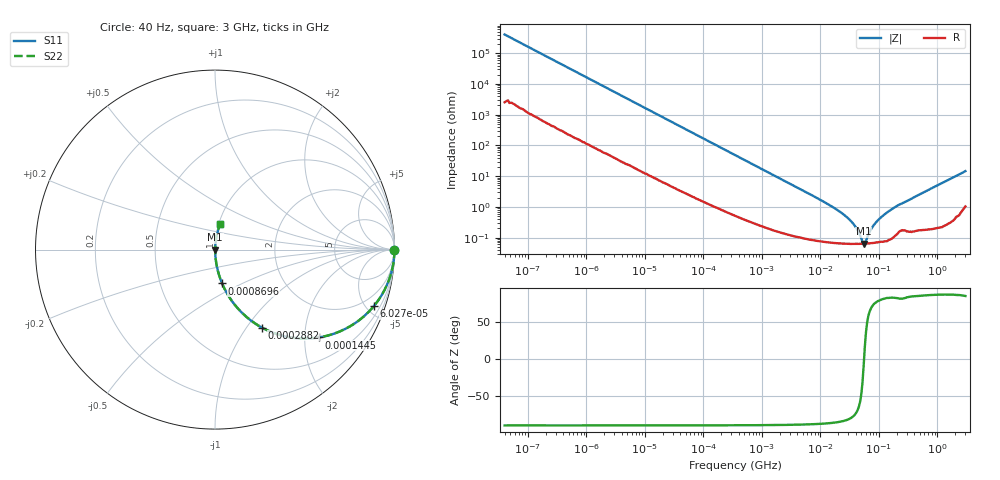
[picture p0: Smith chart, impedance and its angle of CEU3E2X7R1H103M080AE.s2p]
! S-parameter Generated by TDK Corporation
! Copyright(C) 2015 TDK Corporation.
! All Rights Reserved.
! TDK P/N: CEU3E2X7R1H103M080AE (Multilayer Ceramic Chip Capacitors)
! Property: C=10nF
! Size(LxWxT): 1.6x0.8x0.8mm, 0.063x0.031x0.031inches
! Model Type: s2p (Touchstone File Format Version 1.0)
! Frequency: DC=Yes Start=0.00004MHz Stop=3000MHz 396points Log-sweep
! Note: This model was converted from impedance.
! Model Generated on Jun. 23, 2015
! Hash(MD5):
! Port Assignments:
!  1 ---| |--- 2
! Applicable Conditions:
!  Temperature = 25 degC
!  DC Bias Voltage = 0 V
!  Small Signal Operation
! Terms and conditions regarding TDK Simulation Models
! (1)This simulation model is being provided solely for informational purposes. Please refer to the specifications of the products in terms of detailed characteristics of such products.
! (2)In no event shall TDK Corporation of any of its subsidiaries be liable for any loss or damage arising, directly or indirectly,
!  From any information contained in this simulation model, including, but not limited to loss or damages arising from any inaccuracies, omissions or errors in connection with such information.
! (3)Any and all copyrights on this simulation model are owned by TDK Corporation.
!  Duplication or redistribution of this simulation model without prior written permission from TDK Corporation is prohibited.
! (4)This simulation model is subject to any modification or change without any prior notice.
! (5)Neither TDK Corporation nor any of its subsidiaries shall make any warranty, express or implied,
!  Including but not limited to the correctness, implied warranties of merchantability and fitness for a particular purpose with respect to this simulation models.
! (6)The use of this simulation model shall be deemed to have consented to the terms and conditions hereof.
# MHz S MA R 50
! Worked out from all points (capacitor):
!   395 points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, 40 Hz to 3 GHz, reference 50 ohm
!   read as one part in series: C = 9.76 nF near 41.88 Hz
!   lowest |Z| = 64.2 mohm at 54.73 MHz (marker M1)
!   series resonance near 55.61 MHz, so ESL is about 840 pH
!   S11 on the Smith chart (normalised r, x): 40 Hz: open; 60.27 kHz: 1.05, -5.60; 144.5 kHz: 1.02, -2.35; 288.2 kHz: 1.01, -1.18; 869.6 kHz: 1.01, -0.39; 3 GHz: 1.02, +0.29
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4e-05  1 -0.0  0.0002442 89.6  0.0002442 89.6  1 -0.0
0.000834128  1 -0.3  0.005044 89.3  0.005044 89.3  1 -0.3
0.01739424  0.9939 -5.9  0.103 83.7  0.103 83.7  0.9939 -5.9
0.06026525  0.9393 -19.6  0.3353 69.9  0.3353 69.9  0.9393 -19.6
0.09119145  0.8771 -28.2  0.4728 61.3  0.4728 61.3  0.8771 -28.2
0.144487  0.7577 -40.2  0.6458 49.3  0.6458 49.3  0.7577 -40.2
0.2881647  0.5065 -59.0  0.8571 30.4  0.8571 30.4  0.5065 -59.0
0.3464102  0.4397 -63.3  0.8936 26.1  0.8936 26.1  0.4397 -63.3
0.8696408  0.193 -78.1  0.9787 11.1  0.9787 11.1  0.193 -78.1
2.183178  0.07862 -84.5  0.9955 4.5  0.9955 4.5  0.07862 -84.5
7.22376  0.02371 -86.6  0.9989 1.4  0.9989 1.4  0.02371 -86.6
18.13479  0.008661 -85.1  0.9993 0.5  0.9993 0.5  0.008661 -85.1
30.08671  0.004173 -81.1  0.9994 0.2  0.9994 0.2  0.004173 -81.1
41.52283  0.001972 -71.4  0.9994 0.1  0.9994 0.1  0.001972 -71.4
54.72828  0.0006419 -8.8  0.9994 0.0  0.9994 0.0  0.0006419 -8.8
57.30589  0.0006647 16.6  0.9994 -0.0  0.9994 -0.0  0.0006647 16.6
68.88888  0.001509 64.2  0.9993 -0.1  0.9993 -0.1  0.001509 64.2
82.81309  0.002667 75.1  0.9993 -0.1  0.9993 -0.1  0.002667 75.1
104.2405  0.004284 80.0  0.9993 -0.2  0.9993 -0.2  0.004284 80.0
150.6385  0.007467 83.0  0.9991 -0.4  0.9991 -0.4  0.007467 83.0
949.3681  0.04792 84.8  0.9968 -2.7  0.9968 -2.7  0.04792 84.8
3000  0.1435 77.7  0.9795 -8.2  0.9795 -8.2  0.1435 77.7
